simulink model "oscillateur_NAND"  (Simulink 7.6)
settings: Solver=ode15s  StartTime=0.0  StopTime=0.01  RelTol=1e-3
StopFcn:
  | close all, clc
  | load signaux.mat
  | plot(x(1,:),x(2,:))
  | grid
  | title('Oscillateur à portes NAND, T=2RC ln3')
  | 
  | xlabel('temps')
  | axis([0 0.01 -0.1 1.1])
libraries: elec_lib x10, fl_lib x8, nesl_utility x4, gaugeslibv2 x1

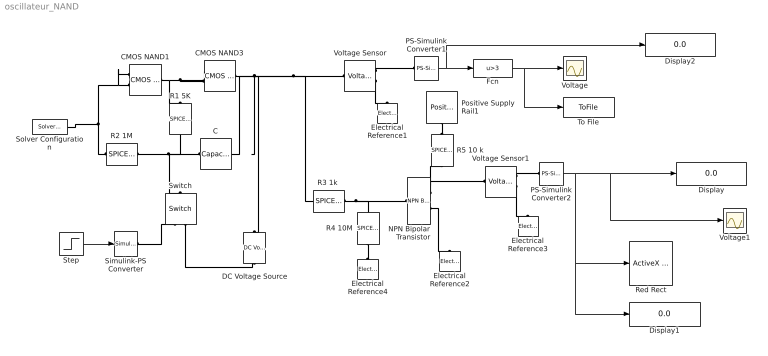
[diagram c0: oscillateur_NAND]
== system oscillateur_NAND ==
  C : fl_lib/Electrical/Electrical Elements/Capacitor  DialogController=NetworkEngine.DynNeDlgSource  SystemSampleTime=-1  c=100e-9 F  v0=0 V  r=1e-6 Ohm  g=0 1/Ohm  i_Log=off  v_Log=off  vc_Log=off  LocalVarNames=|current|voltage|power  LocalVarDescs=|Capacitor current (A)|Voltage across capacitor (V)|Power (W)  LocalVarLogging=[0 0 0]
  CMOS NAND1 : elec_lib/Integrated Circuits/Logic/CMOS NAND  DialogController=NetworkEngine.DynNeDlgSource  SystemSampleTime=-1  V_IL=2 V  V_IH=3 V  C_IN=5 pF  output_type=1  V_OL=0 V  V_OH=5 V  V_CC=5 V  V_meas=5 V  R_OUT=450 Ohm  R_OH=[ 25 250 ] Ohm  I_OH=63 mA  R_OL=[ 30 800 ] Ohm  I_OL=-45 mA  Delay=1.2e-07 s  Ron=5 Ohm  Vf=0.6 V  output_state=1  LocalVarLogging=[]
  CMOS NAND3 : elec_lib/Integrated Circuits/Logic/CMOS NAND  DialogController=NetworkEngine.DynNeDlgSource  SystemSampleTime=-1  V_IL=2 V  V_IH=3 V  C_IN=5 pF  output_type=1  V_OL=0 V  V_OH=5 V  V_CC=5 V  V_meas=5 V  R_OUT=450 Ohm  R_OH=[ 25 250 ] Ohm  I_OH=63 mA  R_OL=[ 30 800 ] Ohm  I_OL=-45 mA  Delay=1.2e-07 s  Ron=5 Ohm  Vf=0.6 V  output_state=1  LocalVarLogging=[]
  DC Voltage Source : elec_lib/Additional Components/SPICE-Compatible Components/Sources/DC Voltage Source  DialogController=NetworkEngine.DynNeDlgSource  SystemSampleTime=-1  DC=1 V  current_Log=off  voltage_Log=off  power_Log=off  LocalVarNames=|current|voltage|power  LocalVarDescs=|Current (A)|Voltage (V)|Power (W)  LocalVarLogging=[0 0 0]
  Display : Display
  Display1 : Display
  Display2 : Display
  Electrical Reference{1..4} (4 alike) : fl_lib/Electrical/Electrical Elements/Electrical Reference  DialogController=NetworkEngine.DynNeDlgSource  SystemSampleTime=-1  i_Log=off  LocalVarNames=|i  LocalVarDescs=|i  LocalVarLogging=[]
  Fcn : Fcn  Expr=u>3
  NPN Bipolar Transistor : elec_lib/Semiconductor Devices/NPN Bipolar Transistor  DialogController=NetworkEngine.DynNeDlgSource  SystemSampleTime=-1  parameterization=1  BF=100  IS=1e-14 A  VAF=200 V  hfe=100  hoe=5e-05 1/Ohm  Ic_h=1 mA  V1=0.55 V  I1=0.5 mA  BR=1  Tmeas=25 C  RC=0.1 Ohm  RE=0.1 Ohm  RB=0.1 Ohm  C_BC=5 pF  C_BE=5 pF  TF=0 us  TR=0 us  LocalVarLogging=[]
  PS-Simulink Converter1 : nesl_utility/PS-Simulink Converter  DialogController=NetworkEngine.DynNeUtilDlgSource  SystemSampleTime=-1  PhysicalDomain=network_engine_domain  LeftPortType=input  RightPortType=output  SubClassName=ps_output  Unit=1  AffineConversion=off
  PS-Simulink Converter2 : nesl_utility/PS-Simulink Converter  DialogController=NetworkEngine.DynNeUtilDlgSource  SystemSampleTime=-1  PhysicalDomain=network_engine_domain  LeftPortType=input  RightPortType=output  SubClassName=ps_output  Unit=1  AffineConversion=off
  Positive Supply Rail1 : elec_lib/Sources/Positive Supply Rail  DialogController=NetworkEngine.DynNeDlgSource  SystemSampleTime=-1  v0=5 V  current_Log=off  voltage_Log=off  power_Log=off  LocalVarNames=|current|voltage|power  LocalVarDescs=|Current (A)|Voltage (V)|Power (W)  LocalVarLogging=[0 0 0]
  R1 5K : elec_lib/Additional Components/SPICE-Compatible Components/Passive Devices/SPICE Resistor  DialogController=NetworkEngine.DynNeDlgSource  SystemSampleTime=-1  SCALE=1  R_param=1  R=5 kOhm  RSH=0 Ohm  LENGTH=1e-06 m  WIDTH=1e-06 m  NARROW=0 m  T_param=1  TC1=0 1/K  TC2=0 1/K^2  TOFFSET=0 K  TFIXED=300.15 K  TMEAS=300.15 K  LocalVarLogging=[]
  R2 1M : elec_lib/Additional Components/SPICE-Compatible Components/Passive Devices/SPICE Resistor  DialogController=NetworkEngine.DynNeDlgSource  SystemSampleTime=-1  SCALE=1  R_param=1  R=1e3 kOhm  RSH=0 Ohm  LENGTH=1e-06 m  WIDTH=1e-06 m  NARROW=0 m  T_param=1  TC1=0 1/K  TC2=0 1/K^2  TOFFSET=0 K  TFIXED=300.15 K  TMEAS=300.15 K  LocalVarLogging=[]
  "R3 1k " : elec_lib/Additional Components/SPICE-Compatible Components/Passive Devices/SPICE Resistor  DialogController=NetworkEngine.DynNeDlgSource  SystemSampleTime=-1  SCALE=1  R_param=1  R=1e3 Ohm  RSH=0 Ohm  LENGTH=1e-06 m  WIDTH=1e-06 m  NARROW=0 m  T_param=1  TC1=0 1/K  TC2=0 1/K^2  TOFFSET=0 K  TFIXED=300.15 K  TMEAS=300.15 K  LocalVarLogging=[]
  R4 10M : elec_lib/Additional Components/SPICE-Compatible Components/Passive Devices/SPICE Resistor  DialogController=NetworkEngine.DynNeDlgSource  SystemSampleTime=-1  SCALE=1  R_param=1  R=10e3 kOhm  RSH=0 Ohm  LENGTH=1e-06 m  WIDTH=1e-06 m  NARROW=0 m  T_param=1  TC1=0 1/K  TC2=0 1/K^2  TOFFSET=0 K  TFIXED=300.15 K  TMEAS=300.15 K  LocalVarLogging=[]
  R5 10 k : elec_lib/Additional Components/SPICE-Compatible Components/Passive Devices/SPICE Resistor  DialogController=NetworkEngine.DynNeDlgSource  SystemSampleTime=-1  SCALE=1  R_param=1  R=10e3 Ohm  RSH=0 Ohm  LENGTH=1e-06 m  WIDTH=1e-06 m  NARROW=0 m  T_param=1  TC1=0 1/K  TC2=0 1/K^2  TOFFSET=0 K  TFIXED=300.15 K  TMEAS=300.15 K  LocalVarLogging=[]
  Red Rect : gaugeslibv2/ActiveX Control  progid=MWLED.ledctrl.1  connect=input  input=Value  init=hActx.configuration='LED\Individual\Red Rectangle';hActx.value=1;hActx.Mode=0;hActx.MouseControl=0;  inblock=on  border=on  updateParam=0
  Simulink-PS Converter : nesl_utility/Simulink-PS Converter  DialogController=NetworkEngine.DynNeUtilDlgSource  SystemSampleTime=-1  PhysicalDomain=network_engine_domain  LeftPortType=input  RightPortType=output  SubClassName=ps_input  Unit=1  AffineConversion=off  InputFilterTimeConstant=.001  UdotUserProvided=0
  Solver Configuration : nesl_utility/Solver Configuration  DialogController=NetworkEngine.DynNeUtilDlgSource  SystemSampleTime=-1  PhysicalDomain=network_engine_domain  LeftPortType=input  RightPortType=generic  SubClassName=solver  Accelerate=off  Profile=off  ResidualTolerance=1e-9  MaxNonlinIter=12  MaxModeIter=2  DoFixedCost=off  UseLocalSampling=off  DoDC=off  LinearAlgebra=Sparse  LocalSolverSampleTime=.001  LocalSolverChoice=NE_BACKWARD_EULER_ADVANCER  UseLocalSolver=off
  Step : Step  Time=0.001  Before=1  After=0  SampleTime=0
  Switch : fl_lib/Electrical/Electrical Elements/Switch  DialogController=NetworkEngine.DynNeDlgSource  SystemSampleTime=-1  R_closed=0.01 Ohm  G_open=1e-08 1/Ohm  Threshold=0  i_Log=off  v_Log=off  LocalVarNames=|i|v  LocalVarDescs=|i|v  LocalVarLogging=[0 0]
  To File : ToFile  Filename=signaux  MatrixName=x
  Voltage : Scope
  Voltage Sensor : fl_lib/Electrical/Electrical Sensors/Voltage Sensor  DialogController=NetworkEngine.DynNeDlgSource  SystemSampleTime=-1  i1_Log=off  v1_Log=off  LocalVarNames=|i1|v1  LocalVarDescs=|i1|v1  LocalVarLogging=[0 0]
  Voltage Sensor1 : fl_lib/Electrical/Electrical Sensors/Voltage Sensor  DialogController=NetworkEngine.DynNeDlgSource  SystemSampleTime=-1  i1_Log=off  v1_Log=off  LocalVarNames=|i1|v1  LocalVarDescs=|i1|v1  LocalVarLogging=[0 0]
  Voltage1 : Scope
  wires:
  Step/1 -> Simulink-PS Converter/1
  PS-Simulink Converter1/1 -> Fcn/1, Display2/1
  Fcn/1 -> Voltage/1, To File/1
  PS-Simulink Converter2/1 -> Red Rect/1, Display1/1, Display/1, Voltage1/1
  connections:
  CMOS NAND1/RConn1 -- CMOS NAND3/LConn1 -- CMOS NAND3/LConn2 -- R1 5K/LConn1
  C/LConn1 -- DC Voltage Source/LConn1 -- CMOS NAND3/RConn1 -- Voltage Sensor/LConn1 -- "R3 1k "/RConn1
  R2 1M/LConn1 -- C/RConn1 -- R1 5K/RConn1 -- Switch/LConn1
  CMOS NAND1/LConn2 -- R2 1M/RConn1 -- Solver Configuration/RConn1 -- CMOS NAND1/LConn1
  Voltage Sensor/RConn2 -- Electrical Reference1/LConn1
  Voltage Sensor/RConn1 -- PS-Simulink Converter1/LConn1
  Switch/RConn2 -- DC Voltage Source/RConn1
  Simulink-PS Converter/RConn1 -- Switch/RConn1
  "R3 1k "/LConn1 -- NPN Bipolar Transistor/LConn1 -- R4 10M/RConn1
  NPN Bipolar Transistor/RConn2 -- Electrical Reference2/LConn1
  NPN Bipolar Transistor/RConn1 -- R5 10 k/LConn1 -- Voltage Sensor1/LConn1
  Positive Supply Rail1/RConn1 -- R5 10 k/RConn1
  Voltage Sensor1/RConn2 -- Electrical Reference3/LConn1
  Voltage Sensor1/RConn1 -- PS-Simulink Converter2/LConn1
  R4 10M/LConn1 -- Electrical Reference4/LConn1
